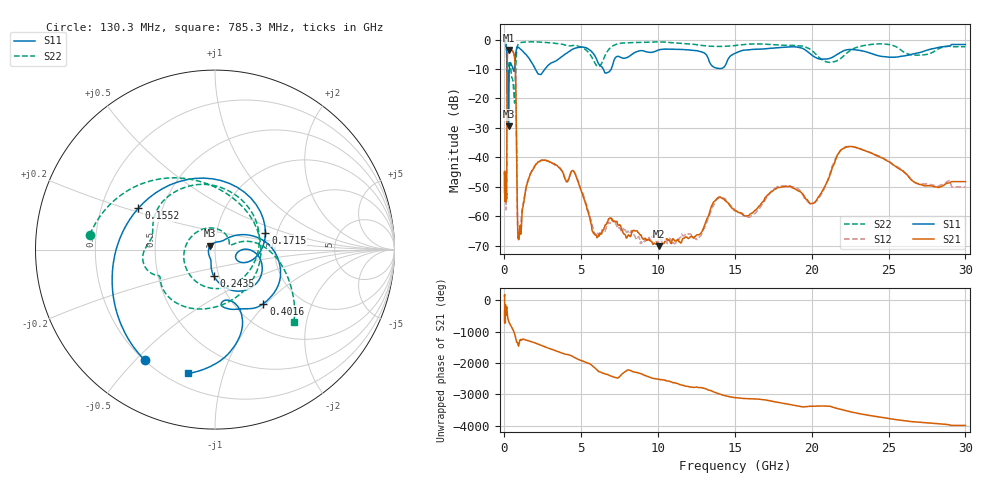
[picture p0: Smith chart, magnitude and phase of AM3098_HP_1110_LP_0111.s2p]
! Date/Time: Thu, Feb 28, 2019 8:46 AM
! Network Analyzer: Agilent Technologies E8364B Rev: A.07.50.67
! Sweep from 0.010 to 30.000 GHz, 1601 Points, Sweep Type: LOG
! Power Supply: 5.022 V, 0.002 A
# Hz S DB R 50
!freq MagS11 AngS11 MagS21 AngS21 MagS12 AngS12 MagS22 AngS22
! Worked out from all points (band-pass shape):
!   1601 points, 10 MHz to 30 GHz, reference 50 ohm
!   highest |S21| = -3.47 dB at 293 MHz (marker M1); lowest = -70.2 dB at 10.08 GHz (marker M2)
!   |S21| within 3 dB of the highest: 183.3 MHz to 665.9 MHz (482.6 MHz wide, 114 % of centre)
!   lowest |S11| = -29.4 dB at 263.8 MHz (marker M3), VSWR 1.07, Z = 47.4 + j2.07 ohm
!   |S11| at or under -10 dB: 170.1 MHz to 317.6 MHz (147.5 MHz wide, 60.5 % of centre); 2.009 GHz to 2.642 GHz (633.2 MHz wide, 27.2 % of centre); 6.431 GHz to 6.947 GHz (515.7 MHz wide, 7.71 % of centre)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
!   |S22| runs from -21.6 to -0.5 dB; largest |S21 - S12| = 0.011
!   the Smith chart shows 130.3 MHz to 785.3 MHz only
!   S11 on the Smith chart (normalised r, x): 130.3 MHz: 0.20, -0.53; 155.2 MHz: 0.37, +0.22; 171.5 MHz: 1.74, +0.35; 243.5 MHz: 0.95, -0.29; 401.6 MHz: 1.34, -0.96; 785.3 MHz: 0.28, -0.77
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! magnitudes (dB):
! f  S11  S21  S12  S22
! 10 MHz  -0.4  -45.4  -45.0  -0.5
! 38.04 MHz  -0.3  -52.2  -51.0  -0.7
! 130.3 MHz  -2.7  -53.4  -54.0  -3.1
! 144.7 MHz  -4.3  -48.8  -50.6  -5.6
! 155.2 MHz  -6.3  -34.4  -34.5  -10.7
! 171.5 MHz  -10.6  -11.6  -11.6  -8.9
! 243.5 MHz  -16.5  -3.8  -3.7  -8.4
! 263.8 MHz  -29.4  -3.5  -3.5  -8.9
! 293 MHz  -14.1  -3.5  -3.4  -8.6
! 401.6 MHz  -7.9  -3.5  -3.5  -9.5
! 550.5 MHz  -9.8  -4.1  -4.1  -14.2
! 703.4 MHz  -6.7  -9.5  -9.5  -15.4
! 785.3 MHz  -3.0  -34.7  -34.6  -4.5
! 921.7 MHz  -2.7  -68.0  -66.9  -1.4
! 2.084 GHz  -10.8  -42.2  -42.2  -0.8
! 4.503 GHz  -3.1  -44.7  -44.6  -2.0
! 5.929 GHz  -5.9  -66.5  -66.1  -8.3
! 7.926 GHz  -6.2  -67.4  -65.5  -1.1
! 10.08 GHz  -3.4  -70.2  -68.1  -0.8
! 20.1 GHz  -5.6  -55.7  -55.6  -4.1
! 22.56 GHz  -3.3  -36.3  -36.3  -3.5
! 30 GHz  -1.6  -48.3  -50.1  -2.4
